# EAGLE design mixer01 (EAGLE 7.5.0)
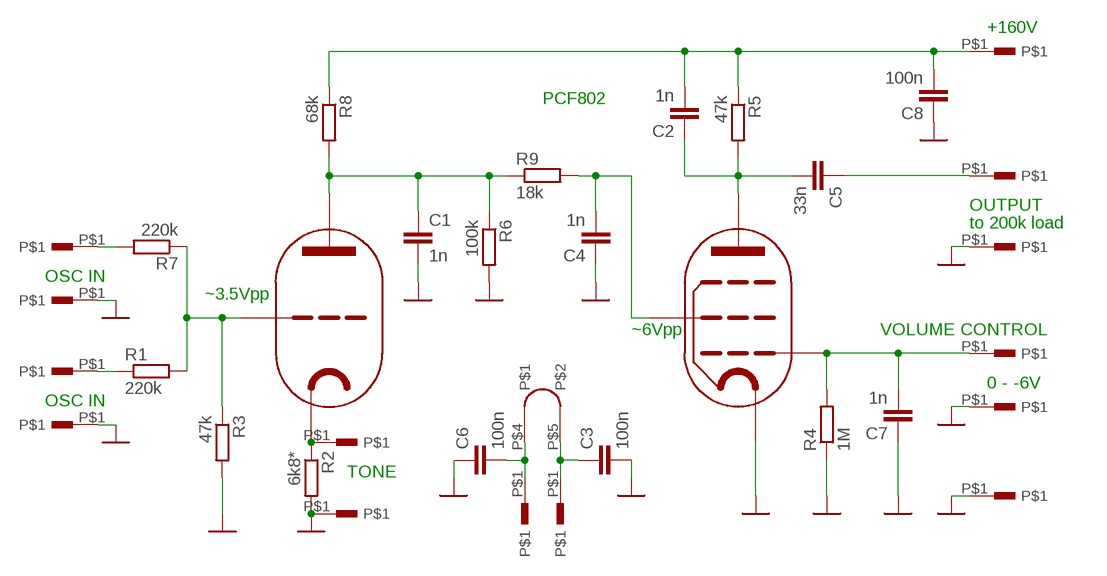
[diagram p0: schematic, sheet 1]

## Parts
C1  1n  C-EU075-032X103  [C075-032X103]
C2  1n  C-EU075-032X103  [C075-032X103]
C3  100n  C-EU050-024X044  [C050-024X044]
C4  1n  C-EU075-032X103  [C075-032X103]
C5  33n  C-EU150-091X182  [C150-091X182]
C6  100n  C-EU050-024X044  [C050-024X044]
C7  1n  C-EU050-024X044  [C050-024X044]
C8  100n  C-EU075-032X103  [C075-032X103]
R1  220k  R-EU_0207/10  [0207/10]
R2  6k8*  R-EU_0207/10  [0207/10]
R3  47k  R-EU_0207/10  [0207/10]
R4  1M  R-EU_0207/10  [0207/10]
R5  47k  R-EU_0207/10  [0207/10]
R6  100k  R-EU_0207/10  [0207/10]
R7  220k  R-EU_0207/10  [0207/10]
R8  68k  R-EU_0207/10  [0207/10]
R9  18k  R-EU_0207/10  [0207/10]
U$1  PCF802  PCF82  [NOVAL02]
U$2  PIN  [PIN]
U$3  PIN  [PIN]
U$4  PIN  [PIN]
U$5  PIN  [PIN]
U$6  PIN  [PIN]
U$7  PIN  [PIN]
U$8  PIN  [PIN]
U$9  PIN  [PIN]
U$10  PIN  [PIN]
U$11  PIN  [PIN]
U$12  PIN  [PIN]
U$13  PIN  [PIN]
U$14  PIN  [PIN]
U$15  PIN  [PIN]

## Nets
GND: C1.2 C3.2 C4.1 C6.1 C7.1 C8.1 R2.2 R3.2 R4.1 R6.2 U$1.P$7(K) U$3.P$1 U$6.P$1 U$9.P$1 U$11.P$1 U$14.P$1 U$15.P$1
N$1: R1.1 U$10.P$1
N$2: C1.1 R6.1 R8.2 R9.1 U$1.P$1(A)
N$3: R2.1 U$1.P$8(K) U$12.P$1
N$4: C2.1 C5.2 R5.2 U$1.P$6(A)
N$5: C2.2 C8.2 R5.1 R8.1 U$4.P$1
N$6: R7.2 U$2.P$1
N$7: R1.2 R3.1 R7.1 U$1.P$9(G1)
N$8: C4.2 R9.2 U$1.P$3(G2)
N$9: C5.1 U$5.P$1
N$10: C6.2 U$1.P$4 U$7.P$1
N$11: C3.1 U$1.P$5 U$8.P$1
N$14: C7.2 R4.2 U$1.P$2(G1) U$13.P$1

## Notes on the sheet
- +160V
- PCF802
- OUTPUT
- to 200k load
- OSC IN
- ~3.5Vpp
- ~6Vpp | VOLUME CONTROL
- 0 - -6V
- OSC IN
- TONE

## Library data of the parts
C1-C8 = rcl:C-EU: CAPACITOR, European symbol
R1-R9 = rcl:R-EU_: RESISTOR, European symbol
U$1 = lampy03:PCF82
U$2-U$15 = lampy04:PIN

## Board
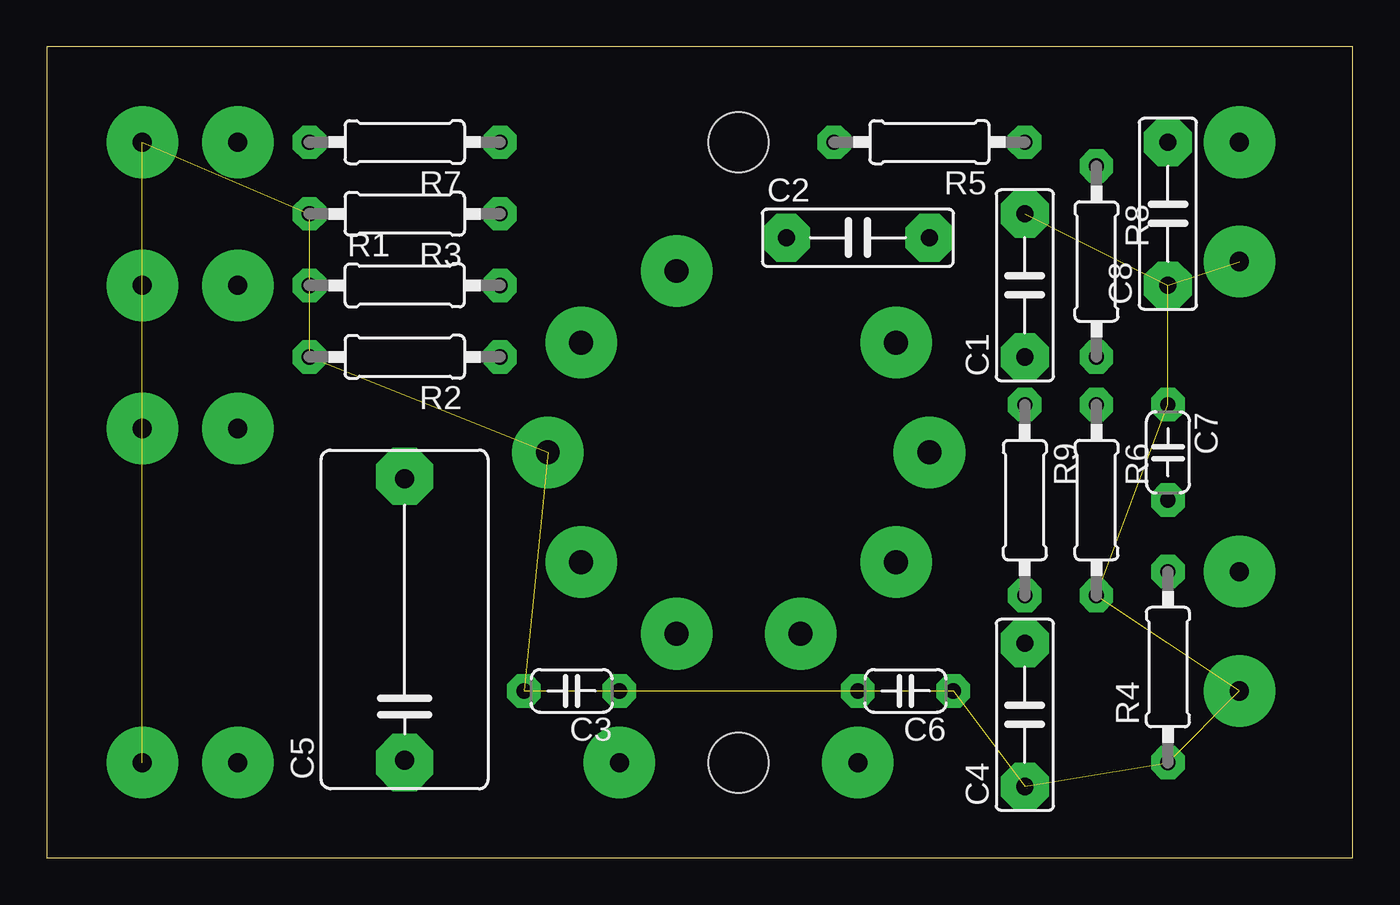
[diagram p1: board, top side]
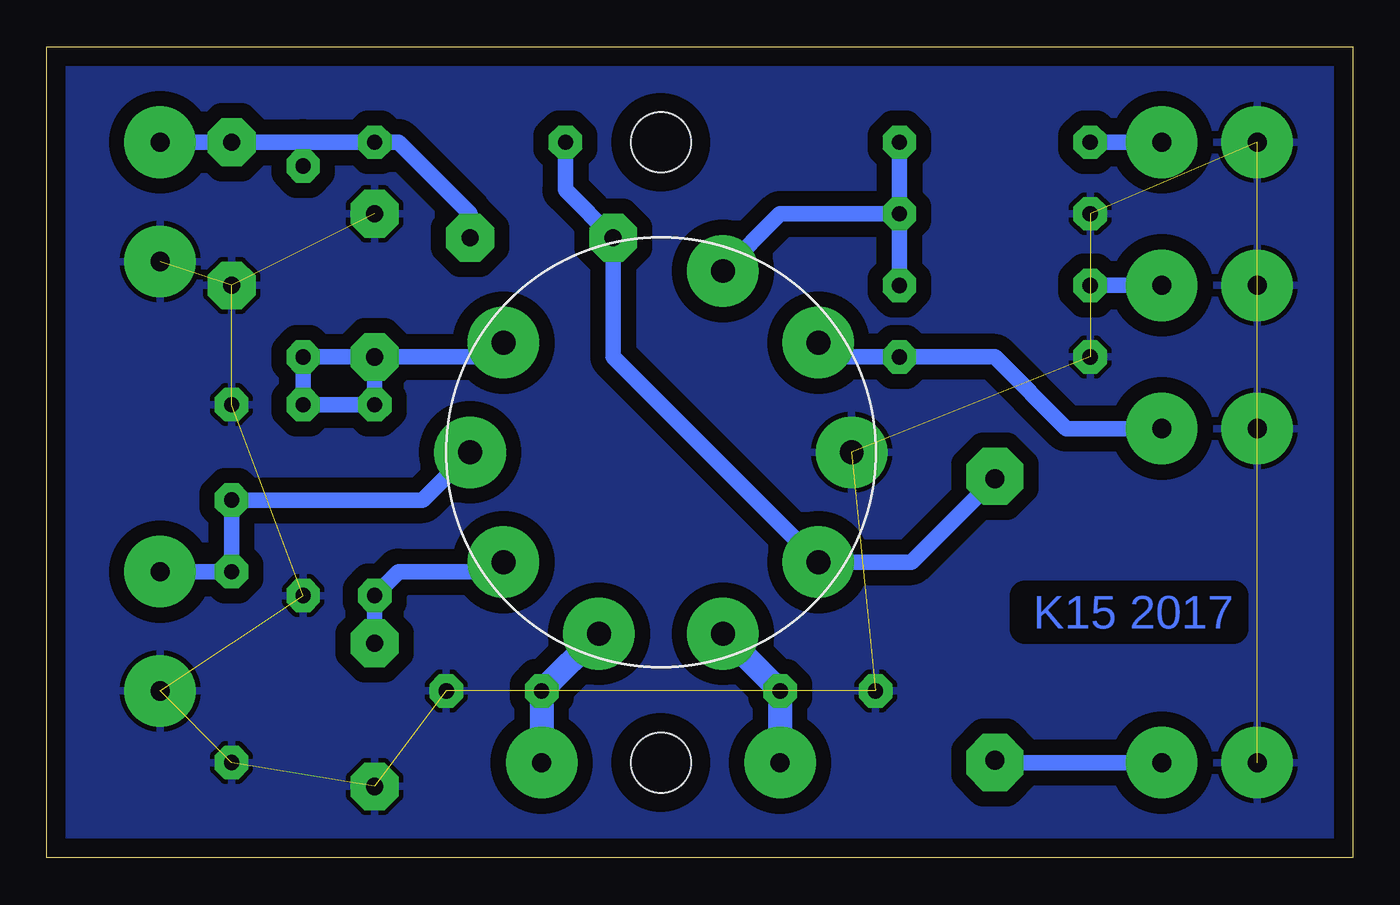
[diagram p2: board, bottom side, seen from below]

Size 69.52 x 43.17 mm. Coordinates in mm from the lower left corner, seen from the top.
Outline: 0,0 69.52,0 69.52,43.17 0,43.17 0,0
Copper layers (1*16): Top 0.035mm / dielectric 1.5mm / Bottom 0.035mm
Design rules "default": minimum track width 10mil, minimum drill 24mil, track to track 8mil, track to pad 8mil, pad to pad 8mil, via to via 8mil, smd to smd 8mil, copper to edge 40mil, drill to drill 8mil, minimum pad ring 10mil, minimum via ring 8mil, stop-mask expansion 4mil, vias tented up to drill 0mil, thermal gap 10mil
Holes 3.2 mm at 36.83,5.08 36.83,38.1

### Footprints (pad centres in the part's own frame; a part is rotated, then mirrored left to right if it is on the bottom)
C075-032X103 = drill 0.914 pad 2.54 octagon: 1 -3.81,0; 2 3.81,0
C050-024X044 = drill 0.813 pad 1.778 octagon: 1 -2.54,0; 2 2.54,0
C150-091X182 = drill 1.016 octagon: 1 -7.493,0; 2 7.493,0
0207/10 = drill 0.813 pad 1.778 octagon: 1 -5.08,0; 2 5.08,0
NOVAL02 = drill 1.27 pad 3.81: P$1 8.382,-5.842; P$2 10.16,0; P$3 8.382,5.842; P$4 3.302,9.652; P$5 -3.302,9.652; P$6 -8.382,5.842; P$7 -10.16,0; P$8 -8.382,-5.842; P$9 -3.302,-9.652
PIN = drill 1.016 pad 3.81: P$1 0,0

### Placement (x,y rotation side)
C1  52.07,30.48 90 top
C2  43.18,33.02 0 top
C3  27.94,8.89 180 top
C4  52.07,7.62 90 top
C5  19.05,12.7 90 top
C6  45.72,8.89 180 top
C7  59.69,21.59 270 top
C8  59.69,34.29 90 top
R1  19.05,30.48 0 top
R2  19.05,26.67 180 top
R3  19.05,34.29 180 top
R4  59.69,10.16 90 top
R5  46.99,38.1 180 top
R6  55.88,19.05 270 top
R7  19.05,38.1 180 top
R8  55.88,31.75 270 top
R9  52.07,19.05 270 top
U$1  36.83,21.59 180 bottom
U$2  10.16,38.1 0 top
U$3  5.08,30.48 0 top
U$4  63.5,38.1 0 top
U$5  10.16,5.08 0 top
U$6  63.5,8.89 0 top
U$7  43.18,5.08 180 top
U$8  30.48,5.08 180 top
U$9  5.08,22.86 0 top
U$10  10.16,30.48 0 top
U$11  5.08,5.08 0 top
U$12  10.16,22.86 0 top
U$13  63.5,15.24 0 top
U$14  63.5,31.75 0 top
U$15  5.08,38.1 0 top

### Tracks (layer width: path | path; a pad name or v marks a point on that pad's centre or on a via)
GND  (16 unrouted)
  pour Bottom (isolate 0.813): 0,43.18 69.85,43.18 69.85,0 0,0
N$1
  Bottom 0.813: U$10.P$1 R1.1
N$2
  Bottom 0.813: C1.1 R8.2 R6.1 R9.1 C1.1 | C1.1 45.72,26.67 U$1.P$1
N$3
  Bottom 0.813: U$1.P$8 27.69,26.67 R2.1 19.05,26.67 15.24,22.86 U$12.P$1
N$4
  Bottom 0.813: C5.2 23.5,15.75 U$1.P$6 39.37,26.67 C2.1 41.91,35.56 R5.2
N$5
  Bottom 0.813: 55.88,38.1 C8.2 U$4.P$1 | 55.88,38.1 R5.1 50.8,38.1 46.99,34.29 C2.2 | R8.1 55.88,38.1
N$6
  Bottom 0.813: U$2.P$1 R7.2
N$7
  Bottom 0.813: R7.1 R3.1 | R1.2 R3.1 | U$1.P$9 30.48,34.29 R3.1
N$8
  Bottom 0.813: U$1.P$3 45.72,15.24 50.8,15.24 R9.2 C4.2
N$9
  Bottom 0.813: U$5.P$1 18.92,5.08 C5.1
N$10
  Bottom 1.27: U$1.P$4 C6.2 U$7.P$1
N$11
  Bottom 1.27: U$1.P$5 C3.1 U$8.P$1
N$12  (via drill 0.6 pad 3.05)
  other vias: 19.05,20.32
N$13  (via drill 0.6 pad 3.05)
  other vias: 19.05,5.08
N$14
  Bottom 0.813: U$13.P$1 R4.2 C7.2 49.53,19.05 U$1.P$2

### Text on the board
Bottom: K15 2017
